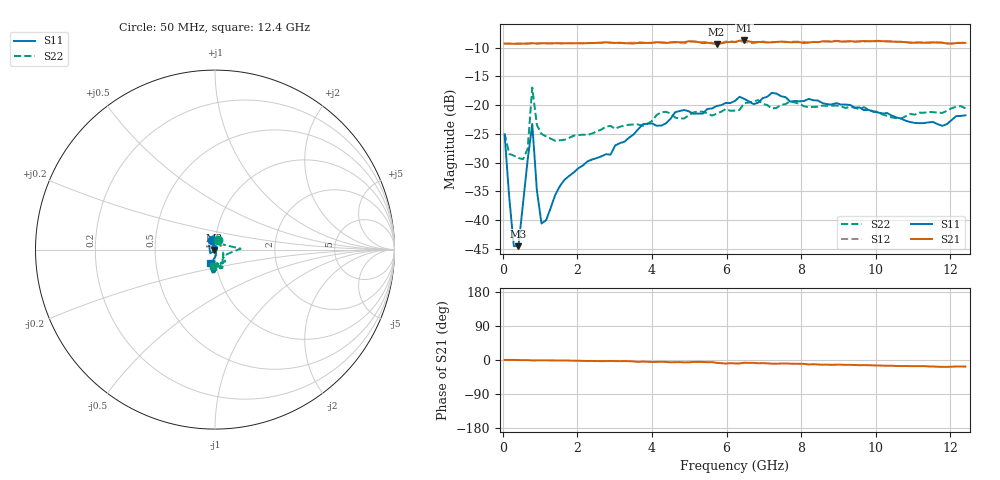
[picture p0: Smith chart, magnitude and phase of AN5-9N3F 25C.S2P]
! Network Analyzer HP8720D.06.14 Serial No. US36140669
! 24 Jul 2008  14:05:50
! Frequency  S11  S21  S12  S22
# HZ  S  DB R 50
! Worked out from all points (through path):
!   101 points, 50 MHz to 12.4 GHz, reference 50 ohm
!   highest |S21| = -8.74 dB at 6.472 GHz (marker M1); lowest = -9.4 dB at 5.731 GHz (marker M2)
!   group delay of S21, straight-line fit = 4.27 ps
!   lowest |S11| = -44.6 dB at 420.5 MHz (marker M3), VSWR 1.01, Z = 49.5 - j0.288 ohm
!   |S11| at or under -10 dB: start of sweep to end of sweep
!   |S22| runs from -29.4 to -16.9 dB; largest |S21 - S12| = 0.011
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5e7  -25.13 109.1  -9.28 0.2  -9.30 -0.0  -24.94 71.5
1.735e8  -36.04 110.0  -9.29 0.1  -9.29 -0.1  -28.49 34.4
2.97e8  -44.54 133.1  -9.32 0.2  -9.30 -0.0  -28.80 26.0
4.205e8  -44.56 -150.6  -9.31 -0.3  -9.28 -0.2  -29.20 24.4
6.675e8  -29.55 -142.8  -9.27 -0.3  -9.29 -0.3  -27.59 51.9
7.91e8  -23.27 123.8  -9.22 -1.2  -9.23 -1.1  -16.94 2.1
9.145e8  -34.78 55.9  -9.28 -1.0  -9.28 -1.0  -23.42 -24.2
1.038e9  -40.61 2.0  -9.23 -1.0  -9.23 -0.9  -25.01 -21.3
1.532e9  -34.09 -73.4  -9.23 -1.2  -9.24 -1.4  -26.12 -22.1
2.1495e9  -30.50 -83.3  -9.24 -2.3  -9.22 -2.1  -25.14 -31.1
2.8905e9  -28.62 -86.1  -9.10 -2.4  -9.15 -2.5  -23.62 -45.1
3.755e9  -23.32 -95.5  -9.16 -4.2  -9.11 -3.5  -23.62 -48.1
4.249e9  -23.56 -96.1  -9.10 -4.6  -9.07 -4.8  -21.23 -51.4
4.6195e9  -21.23 -100.5  -9.00 -5.7  -9.09 -4.9  -22.15 -50.1
5.731e9  -20.16 -99.6  -9.40 -7.5  -9.27 -7.2  -21.50 -68.6
6.225e9  -19.26 -97.4  -9.02 -9.0  -8.98 -7.4  -20.94 -69.9
6.472e9  -18.92 -88.0  -8.74 -7.2  -9.00 -6.7  -19.62 -74.7
7.213e9  -17.86 -96.4  -9.05 -9.7  -9.03 -9.2  -20.59 -68.8
8.3245e9  -19.15 -91.2  -9.01 -11.2  -8.99 -11.0  -20.31 -74.4
1.0424e10  -21.81 -97.3  -8.92 -15.1  -8.92 -15.7  -22.14 -79.5
1.17825e10  -23.60 -108.1  -9.13 -18.1  -9.11 -18.2  -21.36 -95.9
1.24e10  -21.77 -111.4  -9.15 -17.4  -9.12 -17.3  -20.57 -96.0
